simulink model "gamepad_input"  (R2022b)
settings: Solver=FixedStepAuto  StartTime=0.0  StopTime=120  FixedStep=0.001  RelTol=1e-3
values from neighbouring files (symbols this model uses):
  g = 9.8    [compute_quad.m]    (also in compute_quad_lqr_k.m; quad_example.m; quad_example_with_wrapper.m; quad_params.m)
  m = 28/1000    (= 0.028)    [compute_quad.m]    (also in compute_quad_lqr_k.m = 0.0231; quad_example.m; quad_example_with_wrapper.m; quad_params.m)
libraries: vrlib x2

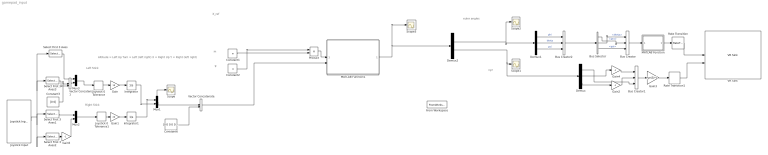
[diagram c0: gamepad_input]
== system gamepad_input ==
  note: g
  note: m
  note: xyz
  note: euler angles
  note: X_ref
  note: Right Stick
  note: Left Stick
  note: Altitude = Left Up Turn = Left (left right) X = Right Up Y = Right (left right)
  Bus Creator : BusCreator  Inputs=3
  Bus Creator1 : BusCreator  Inputs=3
  Bus Creator2 : BusCreator  Inputs=3
  Bus Selector : BusSelector  OutputSignals=phi,theta,psi
  Constant1 : Constant  Value=m
  Constant2 : Constant  Value=g
  Constant3 : Constant  Value=[0 0]  VectorParams1D=off  SampleTime=-1
  Constant6 : Constant  Value=[0 0 0 0 0 0]  VectorParams1D=off  SampleTime=-1
  Demux : Demux  Outputs=3
  Demux1 : Demux  Outputs=3
  Demux2 : Demux  Outputs=2
  From Workspace : FromWorkspace  Commented=on  VariableName=ylogs
  Gain : Gain  Gain=10
  Gain1 : Gain  Gain=20
  Gain2 : Gain  Gain=-1
  Gain3 : Gain  Gain=eye(3)*1  Multiplication=Matrix(K*u)
  Gain4 : Gain  Gain=-1
  Gain5 : Gain  Gain=-1
  Integrator : Integrator
  Integrator1 : Integrator
  Joystick 0 Tolerance : DeadZone  LowerValue=-0.3  UpperValue=0.3
  Joystick 0 Tolerance1 : DeadZone  LowerValue=-0.3  UpperValue=0.3
  Joystick Input : vrlib/Joystick Input  joyid=1  adjustports=on  forcefeed=off
  MATLAB Function : MATLAB Function  TreatAsAtomicUnit=on
  MATLAB Function1 : MATLAB Function  TreatAsAtomicUnit=on
  Mux1 : Mux  Inputs=2
  Mux2 : Mux  Inputs=2
  Mux3 : Mux  Inputs=2
  Product : Product
  Rate Transition : RateTransition  OutPortSampleTime=0.06
  Rate Transition1 : RateTransition  OutPortSampleTime=0.06
  Scope{,1..3} (4 alike) : Scope
  Select First 3 Axes : Selector  InputPortWidth=5  IndexOptions=Index vector (dialog)  Indices=[2]  OutputSizes=1
  Select First 3 Axes1 : Selector  InputPortWidth=5  IndexOptions=Index vector (dialog)  Indices=[5]  OutputSizes=1
  Select First 3 Axes2 : Selector  InputPortWidth=5  IndexOptions=Index vector (dialog)  Indices=[4]  OutputSizes=1
  Select First 3 Axes3 : Selector  InputPortWidth=5  IndexOptions=Index vector (dialog)  Indices=[1]  OutputSizes=1
  VR Sink : vrlib/VR Sink  InstantiateOnLoad=on  SampleTime=-1  ViewEnable=on  RemoteChange=off  RemoteView=off  FieldsWritten=Helicopter.rotation.4.1.1.double#Helicopter.translation.3.1.1.double  WorldFileName=quadrotor_world_ucart.wrl  AutoView=on  VideoDimensions=[]  AllowVariableSize=off
  Vector Concatenate : Concatenate
  Vector Concatenate1 : Concatenate
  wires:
  Rate Transition1/1 -> VR Sink/2
  Bus Selector/2 -> Bus Creator/1  "<theta>"
  Demux1/1 -> Bus Creator2/1  "phi"
  MATLAB Function/1(y) -> Rate Transition/1
  Bus Creator/1 -> MATLAB Function/1(u)
  Demux1/2 -> Bus Creator2/2  "theta"
  Demux1/3 -> Bus Creator2/3  "psi"
  Demux/3 -> Gain2/1
  Gain3/1 -> Rate Transition1/1
  Bus Creator2/1 -> Bus Selector/1
  Gain2/1 -> Bus Creator1/2
  Bus Creator1/1 -> Gain3/1
  Gain4/1 -> Bus Creator1/1
  Demux/1 -> Bus Creator1/3
  Demux/2 -> Gain4/1
  Rate Transition/1 -> VR Sink/1
  Demux2/2 -> Demux/1, Scope1/1
  Demux2/1 -> Scope2/1, Demux1/1
  Product/1 -> MATLAB Function1/1(F_hover)
  Constant1/1 -> Product/2
  Constant2/1 -> Product/1
  Joystick 0 Tolerance/1 -> Gain/1
  Mux1/1 -> Scope/1, Vector Concatenate/1
  Joystick Input/1 -> Select First 3 Axes2/1, Select First 3 Axes1/1, Select First 3 Axes3/1, Select First 3 Axes/1
  Gain1/1 -> Integrator1/1
  Gain/1 -> Integrator/1
  Joystick 0 Tolerance1/1 -> Gain1/1
  Integrator1/1 -> Mux1/1
  Constant6/1 -> Vector Concatenate/2
  Vector Concatenate/1 -> MATLAB Function1/2(X_ref)
  Select First 3 Axes2/1 -> Gain5/1
  Gain5/1 -> Mux2/2
  Select First 3 Axes1/1 -> Mux2/1
  Mux2/1 -> Joystick 0 Tolerance1/1
  MATLAB Function1/1(outputs) -> Demux2/1, Scope3/1
  Bus Selector/1 -> Bus Creator/2  "<phi>"
  Bus Selector/3 -> Bus Creator/3  "<psi>"
  Integrator/1 -> Mux1/2
  Vector Concatenate1/1 -> Mux3/2
  Select First 3 Axes/1 -> Mux3/1
  Mux3/1 -> Joystick 0 Tolerance/1
  Constant3/1 -> Vector Concatenate1/1
  Select First 3 Axes3/1 -> Vector Concatenate1/2

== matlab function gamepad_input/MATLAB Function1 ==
function outputs = fcn(F_hover, X_ref)

coder.extrinsic('evalin', 'assignin')

Xsize = 20;

Xsize = evalin('base', 'Xsize');

X = zeros(Xsize,12);
U = zeros(1, 4);
tspan = zeros(1, 2);

X = evalin('base', 'X');
U = evalin('base', 'U');
tspan = evalin('base', 'tspan');


tspan=[tspan(2) tspan(2)+0.001];

outputs = zeros(1, 6);
[outputs, Xrot, Urot, tspanout] = compute_quad_wrapper(0.001, X, U, X_ref, F_hover, tspan);

assignin('base', 'X', Xrot);
assignin('base', 'U', Urot);
assignin('base', 'tspan', tspanout);
assignin('base', 'Xsize', size(Xrot,1))


end

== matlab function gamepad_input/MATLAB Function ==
function y = eigenaxis_ucart(u)


if abs(u(1))< 0.0001
    u(1) = 0.0001;
end

if abs(u(2))< 0.0001
    u(2) = 0.0001;
end

if abs(u(3))< 0.0001
    u(3) = 0.0001;
end

u = [ -u(1); -u(2); u(3) ];% [Pitch, Yaw, Roll] 

C11 = cos(u(2))*cos(u(3));
C12 = cos(u(2))*sin(u(3));
C13 = -sin(u(2));
C21 = sin(u(1))*sin(u(2))*cos(u(3))-cos(u(1))*sin(u(3));
C22 = sin(u(1))*sin(u(2))*sin(u(3))+cos(u(1))*cos(u(3));
C23 = sin(u(1))*cos(u(2));
C31 = cos(u(1))*sin(u(2))*cos(u(3))+sin(u(1))*sin(u(3));
C32 = cos(u(1))*sin(u(2))*sin(u(3))-sin(u(1))*cos(u(3));
C33 = cos(u(1))*cos(u(2));
    
theta = acos(0.5*(C11+C22+C33-1));

e = [C23-C32; C31-C13; C12-C21]/(2*sin(theta));
    
y = [e; theta];
